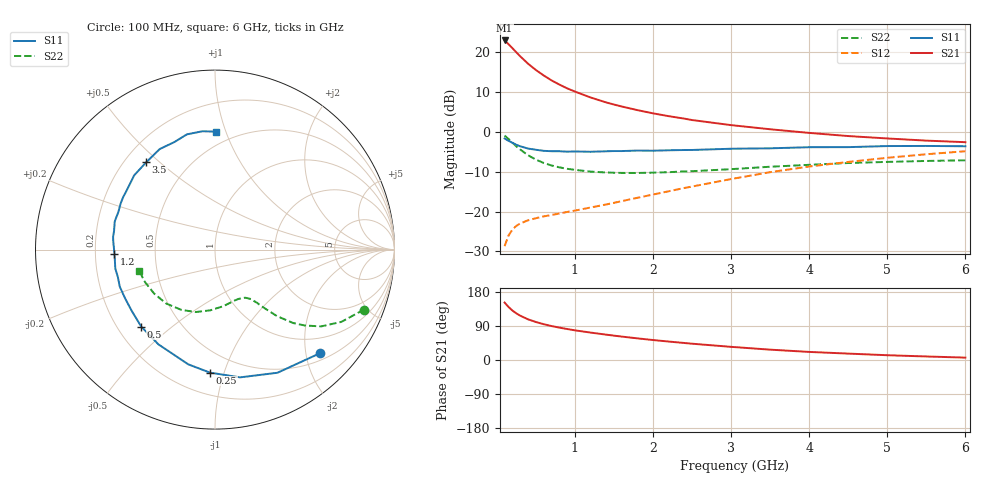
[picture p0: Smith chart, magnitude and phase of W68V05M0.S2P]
! SIEMENS Small Signal Semiconductors
! BFR193W
! Si NPN RF Bipolar Junction Transistor in SOT323
! VCE = 8 V  IC = 5 mA
! Common Emitter S-Parameters:  September  1992
# GHz  S  MA  R  50
!  f  S11  S21  S12  S22
! GHz  MAG  ANG  MAG  ANG  MAG  ANG  MAG  ANG
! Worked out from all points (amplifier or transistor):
!   28 points, 100 MHz to 6 GHz, reference 50 ohm
!   highest |S21| = 22.9 dB at 100 MHz (marker M1)
!   |S21| within 3 dB of that: start of sweep to 251.7 MHz
!   unconditionally stable (mu >= 1): 1.21 GHz to 2.593 GHz
!   at 300 MHz: K = 0.36, MSG = 20.9 dB, |S12| = -23.0 dB
!   at 1.5 GHz: K = 1.05, MAG = 10.9 dB, |S12| = -17.8 dB
!   at 6 GHz: K = 0.89, MSG = 1.1 dB, |S12| = -4.9 dB
!   lowest NFmin = 1.20 dB at 450 MHz
!   S11 on the Smith chart (normalised r, x): 100 MHz: 0.64, -2.29; 250 MHz: 0.35, -0.90; 500 MHz: 0.30, -0.39; 1.2 GHz: 0.28, -0.02; 3.5 GHz: 0.29, +0.45; 6 GHz: 0.40, +0.93
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0.1  0.8225 -44.5  13.91 151.5  0.0368 67.6  0.8954 -21.9
0.15  0.7694 -63.1  12.49 139.9  0.05 59.5  0.8106 -29.8
0.2  0.7254 -78.9  11.13 130.5  0.0593 53.4  0.7298 -35.9
0.25  0.6858 -92.4  9.883 123.1  0.0661 49.0  0.6553 -40.2
0.3  0.6564 -103.1  8.799 116.9  0.0709 46.0  0.5978 -43.2
0.4  0.615 -120.8  7.116 107.3  0.0776 42.7  0.507 -47.0
0.5  0.5941 -133.8  5.934 100.3  0.0824 41.6  0.4474 -49.0
0.6  0.5759 -143.8  5.069 94.5  0.0869 41.7  0.4056 -50.7
0.7  0.5697 -151.8  4.397 89.6  0.0905 42.5  0.3779 -51.7
0.8  0.5693 -158.7  3.901 85.5  0.0943 43.9  0.3578 -52.9
0.9  0.5624 -164.2  3.495 81.8  0.0987 45.4  0.3429 -53.7
1  0.5654 -169.2  3.184 78.3  0.1027 47.1  0.3328 -55.1
1.2  0.5605 -177.6  2.685 72.4  0.1122 50.3  0.3162 -57.9
1.4  0.5686 175.5  2.328 66.9  0.1226 53.3  0.3084 -61.1
1.6  0.5721 169.3  2.069 61.8  0.1349 56.1  0.3045 -64.6
1.8  0.5802 164.3  1.864 57.1  0.1486 58.4  0.304 -68.7
2.2  0.5851 154.0  1.566 48.7  0.1793 61.5  0.311 -76.7
3  0.6117 137.4  1.209 34.7  0.2552 62.6  0.3394 -94.5
3.5  0.6192 128.3  1.073 27.3  0.3112 60.3  0.364 -107.1
4.5  0.6406 110.6  0.882 16.9  0.418 52.3  0.4053 -132.2
5.5  0.6631 96.0  0.773 9.3  0.5217 42.6  0.43 -155.2
6  0.657 89.5  0.739 6.3  0.5694 37.0  0.4383 -163.9
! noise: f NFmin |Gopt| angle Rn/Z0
0.45  1.2  0.26  102  0.14
0.9  1.25  0.38  145  0.12
1.8  2.05  0.56  -161  0.12
